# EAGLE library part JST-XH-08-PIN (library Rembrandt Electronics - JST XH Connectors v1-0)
JST XH Connector 2 Pin Wire to board connector. Pitch: 2,54 mm, (0.100") Number of pins: 8 Created by Rembrandt Electronics www.rembrandtelectronics.com
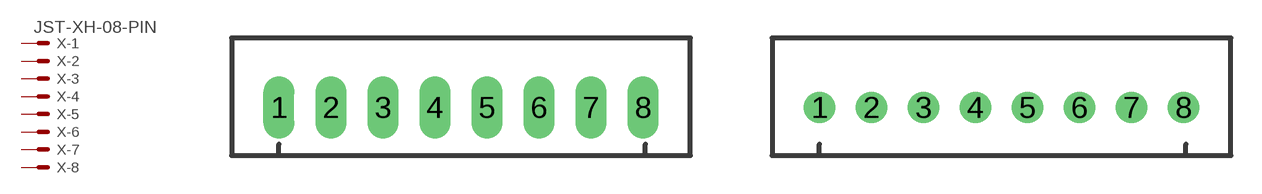
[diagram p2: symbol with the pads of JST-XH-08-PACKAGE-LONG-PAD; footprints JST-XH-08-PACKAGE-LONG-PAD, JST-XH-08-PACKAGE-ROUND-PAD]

Designator prefix X; gates -1=MV -2=M -3=M -4=M -5=M -6=M -7=M -8=M

## JST-XH-08-PIN-LONG-PAD  [JST-XH-08-PACKAGE-LONG-PAD]
1  -1:S  pas
2  -2:S  pas
3  -3:S  pas
4  -4:S  pas
5  -5:S  pas
6  -6:S  pas
7  -7:S  pas
8  -8:S  pas

## JST-XH-08-PIN-ROUND-PAD  [JST-XH-08-PACKAGE-ROUND-PAD]
Pads as for JST-XH-08-PACKAGE-LONG-PAD

## Footprint JST-XH-08-PACKAGE-LONG-PAD (pad centres in mm)
JST XH Connector Long Pads (Package) Wire to board connector. Pitch: 2,54 mm, (0.100") Number of pins: 8 Created by Rembrandt Electronics www.rembrandtelectronics.com
drill 1.016 long: 1 -8.89,0; 2 -6.35,0; 3 -3.81,0; 4 -1.27,0; 5 1.27,0; 6 3.81,0; 7 6.35,0; 8 8.89,0

## Footprint JST-XH-08-PACKAGE-ROUND-PAD (pad centres in mm)
JST XH Connector Round Pads (Package) Wire to board connector. Pitch: 2,54 mm, (0.100") Number of pins: 8 Created by Rembrandt Electronics www.rembrandtelectronics.com
drill 1.016: 1 -8.89,0; 2 -6.35,0; 3 -3.81,0; 4 -1.27,0; 5 1.27,0; 6 3.81,0; 7 6.35,0; 8 8.89,0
